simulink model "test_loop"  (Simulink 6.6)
settings: Solver=ode45  StartTime=0.0  StopTime=10.0  RelTol=1e-3
libraries: sltpda x13

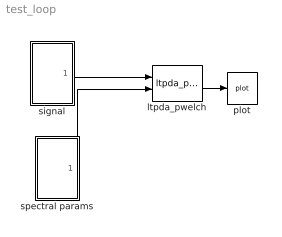
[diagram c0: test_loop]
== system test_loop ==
  ltpda_pwelch : sltpda/Signal Processing blocks/Frequency domain/ltpda_pwelch  Tag=ltpda_pwelch  Description=Makes a spectral density estimate by calling ltpda_pwlech.  SystemSampleTime=-1  win=Hanning  nfft=1000
  plot : sltpda/Sinks/plot  Tag=plot  Description=Plot an analysis object.  SystemSampleTime=-1  xscale=linear  yscale=linear
  signal : Subsystem
  spectral params : Subsystem
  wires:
  signal/1(Out1) -> ltpda_pwelch/1
  ltpda_pwelch/1 -> plot/1
  spectral params/1(Out1) -> ltpda_pwelch/2

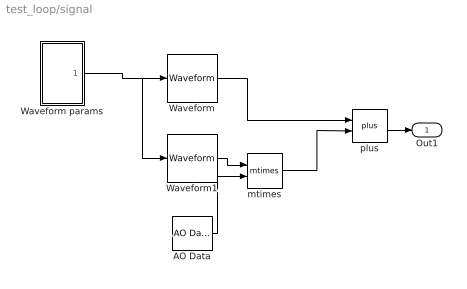
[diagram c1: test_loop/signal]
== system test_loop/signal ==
  AO Data : sltpda/Sources/AO Data  Tag=ao  SystemSampleTime=-1  vals=0.01
  Waveform : sltpda/Sources/Waveform  SystemSampleTime=-1  waveform=Square wave  freq=30  phi=0  ntype=Normal  chirp_f0=10  chirp_fe=400  chirp_te=10  gp_f0=0  gp_bw=0  square_duty=50  sawtooth_width=0
  Waveform params : Subsystem
  Waveform1 : sltpda/Sources/Waveform  SystemSampleTime=-1  waveform=noise  freq=0  phi=0  ntype=Normal  chirp_f0=0  chirp_fe=0  chirp_te=0  gp_f0=0  gp_bw=0  square_duty=0  sawtooth_width=0
  mtimes : sltpda/math blocks/mtimes  Tag=mtimes  SystemSampleTime=-1
  plus : sltpda/math blocks/plus  Tag=plus  SystemSampleTime=-1
  Out1 : Outport
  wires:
  Waveform params/1(Out1) -> Waveform/1, Waveform1/1
  Waveform/1 -> plus/1
  Waveform1/1 -> mtimes/1
  AO Data/1 -> mtimes/2
  mtimes/1 -> plus/2
  plus/1 -> Out1/1

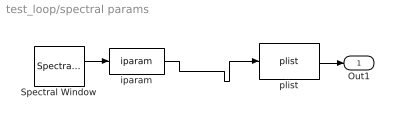
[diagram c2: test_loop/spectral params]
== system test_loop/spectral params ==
  Spectral Window : sltpda/Sources/Spectral Window  Tag=specwin  SystemSampleTime=-1  wname=Kaiser  wlen=1  psll=200
  iparam : sltpda/Parameters/iparam  Tag=iparam  SystemSampleTime=-1  key=Win
  plist : sltpda/Parameters/plist  SystemSampleTime=-1
  Out1 : Outport
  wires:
  Spectral Window/1 -> iparam/1
  plist/1 -> Out1/1
  iparam/1 -> plist/1

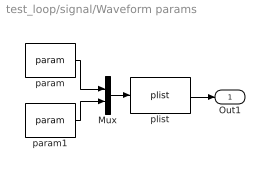
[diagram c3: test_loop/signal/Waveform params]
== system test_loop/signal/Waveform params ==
  Mux : Mux  Inputs=2
  param : sltpda/Parameters/param  Tag=param  SystemSampleTime=-1  key=nsecs  value=10
  param1 : sltpda/Parameters/param  Tag=param  SystemSampleTime=-1  key=fs  value=1000
  plist : sltpda/Parameters/plist  SystemSampleTime=-1
  Out1 : Outport
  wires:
  param/1 -> Mux/1
  param1/1 -> Mux/2
  Mux/1 -> plist/1
  plist/1 -> Out1/1
